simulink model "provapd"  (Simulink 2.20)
settings: Solver=ode45  StartTime=0.0  StopTime=10.0  RelTol=1e-3  AbsTol=1e-6

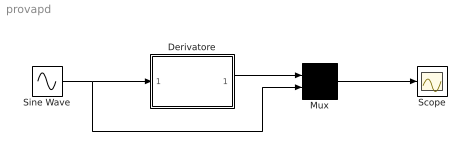
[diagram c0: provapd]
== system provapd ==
  Derivatore : Subsystem  mask(Simulazione Derivatore implementato in maniera software){Td=1, T=0.130, N=10}
      mask prompts: Td "Costante di derivazione Td"; T "Sample Time T del PD"; N "Indice polo del derivatore [5..10]"
      mask init:
      | Kbeta=Td/(N*T+Td);
      | Kalfa=N*Kbeta;
  Mux : Mux  Inputs=2
  Scope : Scope
  Sine Wave : Sin  Amplitude=15  Frequency=1  Phase=0  SampleTime=0
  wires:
  Mux/1 -> Scope/1
  Derivatore/1(Out1) -> Mux/1
  Sine Wave/1 -> Derivatore/1(In1), Mux/2

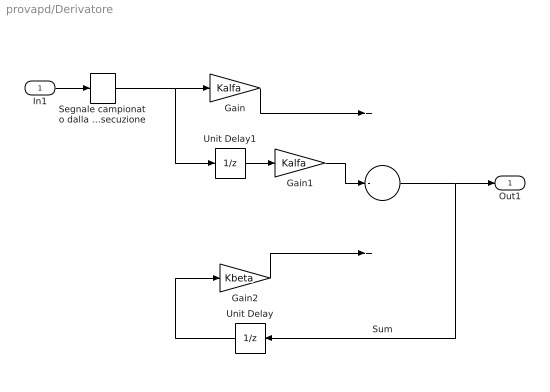
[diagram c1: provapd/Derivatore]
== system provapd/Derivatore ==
  In1 : Inport  Port=1  PortWidth=-1  SampleTime=-1
  Gain : Gain  Gain=Kalfa
  Gain1 : Gain  Gain=Kalfa
  Gain2 : Gain  Gain=Kbeta
  Segnale campionato dalla procedura software al momento del ciclo  d 'esecuzione : ZeroOrderHold  SampleTime=T
  Sum : Sum  Inputs=+-+
  Unit Delay : UnitDelay  Orientation=left  X0=0  SampleTime=T
  Unit Delay1 : UnitDelay  X0=0  SampleTime=T
  Out1 : Outport  Port=1
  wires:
  Gain1/1 -> Sum/2
  Unit Delay/1 -> Gain2/1
  Gain2/1 -> Sum/3
  Gain/1 -> Sum/1
  Unit Delay1/1 -> Gain1/1
  Sum/1 -> Out1/1, Unit Delay/1
  In1/1 -> Segnale campionato dalla procedura software al momento del ciclo  d 'esecuzione/1
  Segnale campionato dalla procedura software al momento del ciclo  d 'esecuzione/1 -> Gain/1, Unit Delay1/1
